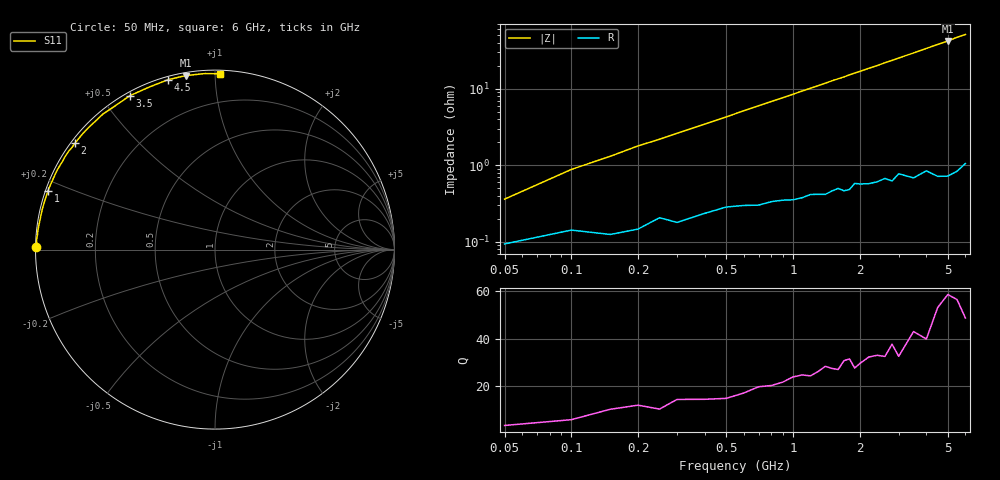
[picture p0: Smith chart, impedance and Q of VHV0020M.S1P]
! Infineon Technologies  Discrete & RF Semiconductors
! BB 814
! Si Tuning Diode in SOT23
! VR =
! S-Parameters:  July  1999
# GHz  S  MA  R  50
!  f  S11
! GHz  MAG  ANG
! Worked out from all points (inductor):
!   34 points, 50 MHz to 6 GHz, reference 50 ohm
!   read as one part to ground: L = 1.39 nH near 50 MHz
!   highest Q = 56.3 at 5 GHz (marker M1), where L = 1.34 nH
!   S11 on the Smith chart (normalised r, x): 50 MHz: 0.00, +0.01; 1 GHz: 0.01, +0.17; 2 GHz: 0.01, +0.34; 3.5 GHz: 0.01, +0.59; 4.5 GHz: 0.01, +0.76; 6 GHz: 0.02, +1.03
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0.05  0.9962 179.2
0.1  0.9943 178.0
0.2  0.9941 175.9
0.25  0.9918 175.0
0.4  0.9907 172.1
0.7  0.9882 166.3
0.8  0.9869 164.4
1  0.9863 160.7
1.1  0.9855 158.8
1.3  0.9842 155.2
1.4  0.9843 153.3
1.5  0.9828 151.4
1.6  0.9816 149.7
1.7  0.9829 148.0
1.8  0.9825 146.1
1.9  0.9791 144.3
2  0.9797 142.7
2.2  0.98 139.2
2.4  0.9792 136.1
2.6  0.9776 132.6
2.8  0.9798 129.6
3  0.9756 126.3
3.5  0.9798 119.0
4  0.977 111.9
4.5  0.982 105.4
5  0.9833 99.6
5.5  0.9824 93.3
6  0.9797 88.4
